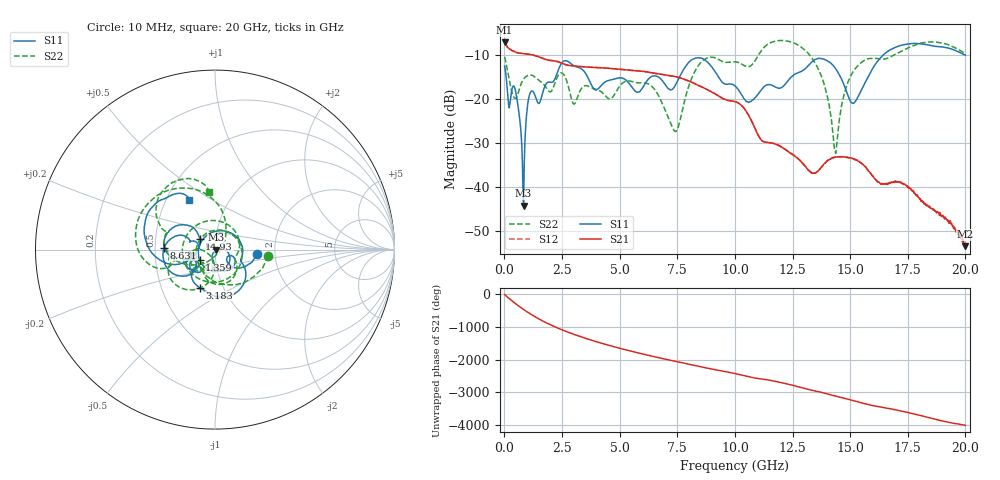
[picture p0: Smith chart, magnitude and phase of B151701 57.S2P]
!  2-Port S-parameters saved by WinCal
! VAR MeasName=S-Parameters (CALIBRATED_DATA) read from VNA (N5244A)
! VAR MeasDate=2015-12-24 19:16:44
! VAR NAME=B151701 57
! VAR FILENAME=B151701 57.S2P
! VAR DATE=2015-12-24 19:16:44
! VAR PHYS_PORTS=1,3
# Hz S DB R 50
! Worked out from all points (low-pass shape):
!   801 points, 10 MHz to 20 GHz, reference 50 ohm
!   highest |S21| = -7.16 dB at 10 MHz (marker M1); lowest = -53.5 dB at 20 GHz (marker M2)
!   |S21| within 3 dB of the highest: start of sweep to 1.307 GHz
!   lowest |S11| = -44.3 dB at 834.6 MHz (marker M3), VSWR 1.01, Z = 50.6 - j0.0944 ohm
!   |S11| at or under -10 dB: start of sweep to 16.45 GHz; 19.97237 GHz to end of sweep
!   |S22| runs from -32.4 to -6.7 dB; largest |S21 - S12| = 0.0011
!   S11 on the Smith chart (normalised r, x): 10 MHz: 1.61, -0.09; 1.359 GHz: 0.84, -0.10; 3.183 GHz: 0.78, -0.35; 8.631 GHz: 0.56, +0.01; 14.93 GHz: 0.84, +0.10; 20 GHz: 0.65, +0.40
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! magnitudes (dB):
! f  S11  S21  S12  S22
! 10 MHz  -12.5  -7.2  -7.1  -10.5
! 209.9 MHz  -22.1  -8.6  -8.6  -15.7
! 509.8 MHz  -18.9  -9.4  -9.4  -19.8
! 834.6 MHz  -44.3  -9.7  -9.7  -15.5
! 1.059 GHz  -19.8  -9.9  -9.9  -14.6
! 1.359 GHz  -19.7  -10.2  -10.2  -15.2
! 2.509 GHz  -11.7  -11.9  -11.9  -14.2
! 3.183 GHz  -12.8  -12.6  -12.6  -19.5
! 3.358 GHz  -13.2  -12.7  -12.7  -17.6
! 3.958 GHz  -18.0  -12.9  -12.9  -17.9
! 6.682 GHz  -15.1  -14.3  -14.3  -19.2
! 7.456 GHz  -16.5  -15.0  -15.0  -27.4
! 8.631 GHz  -11.0  -17.5  -17.5  -11.2
! 10.01 GHz  -17.1  -20.6  -20.6  -11.6
! 10.65 GHz  -20.6  -24.3  -24.3  -12.6
! 11.9 GHz  -17.6  -30.6  -30.6  -6.8
! 13.35 GHz  -11.6  -36.8  -36.7  -10.8
! 13.93 GHz  -11.2  -34.6  -34.4  -17.8
! 14.35 GHz  -13.0  -33.3  -33.2  -32.1
! 14.93 GHz  -19.6  -33.4  -33.4  -15.9
! 16.68 GHz  -9.1  -39.3  -39.1  -10.7
! 20 GHz  -10.1  -53.5  -53.3  -9.8
